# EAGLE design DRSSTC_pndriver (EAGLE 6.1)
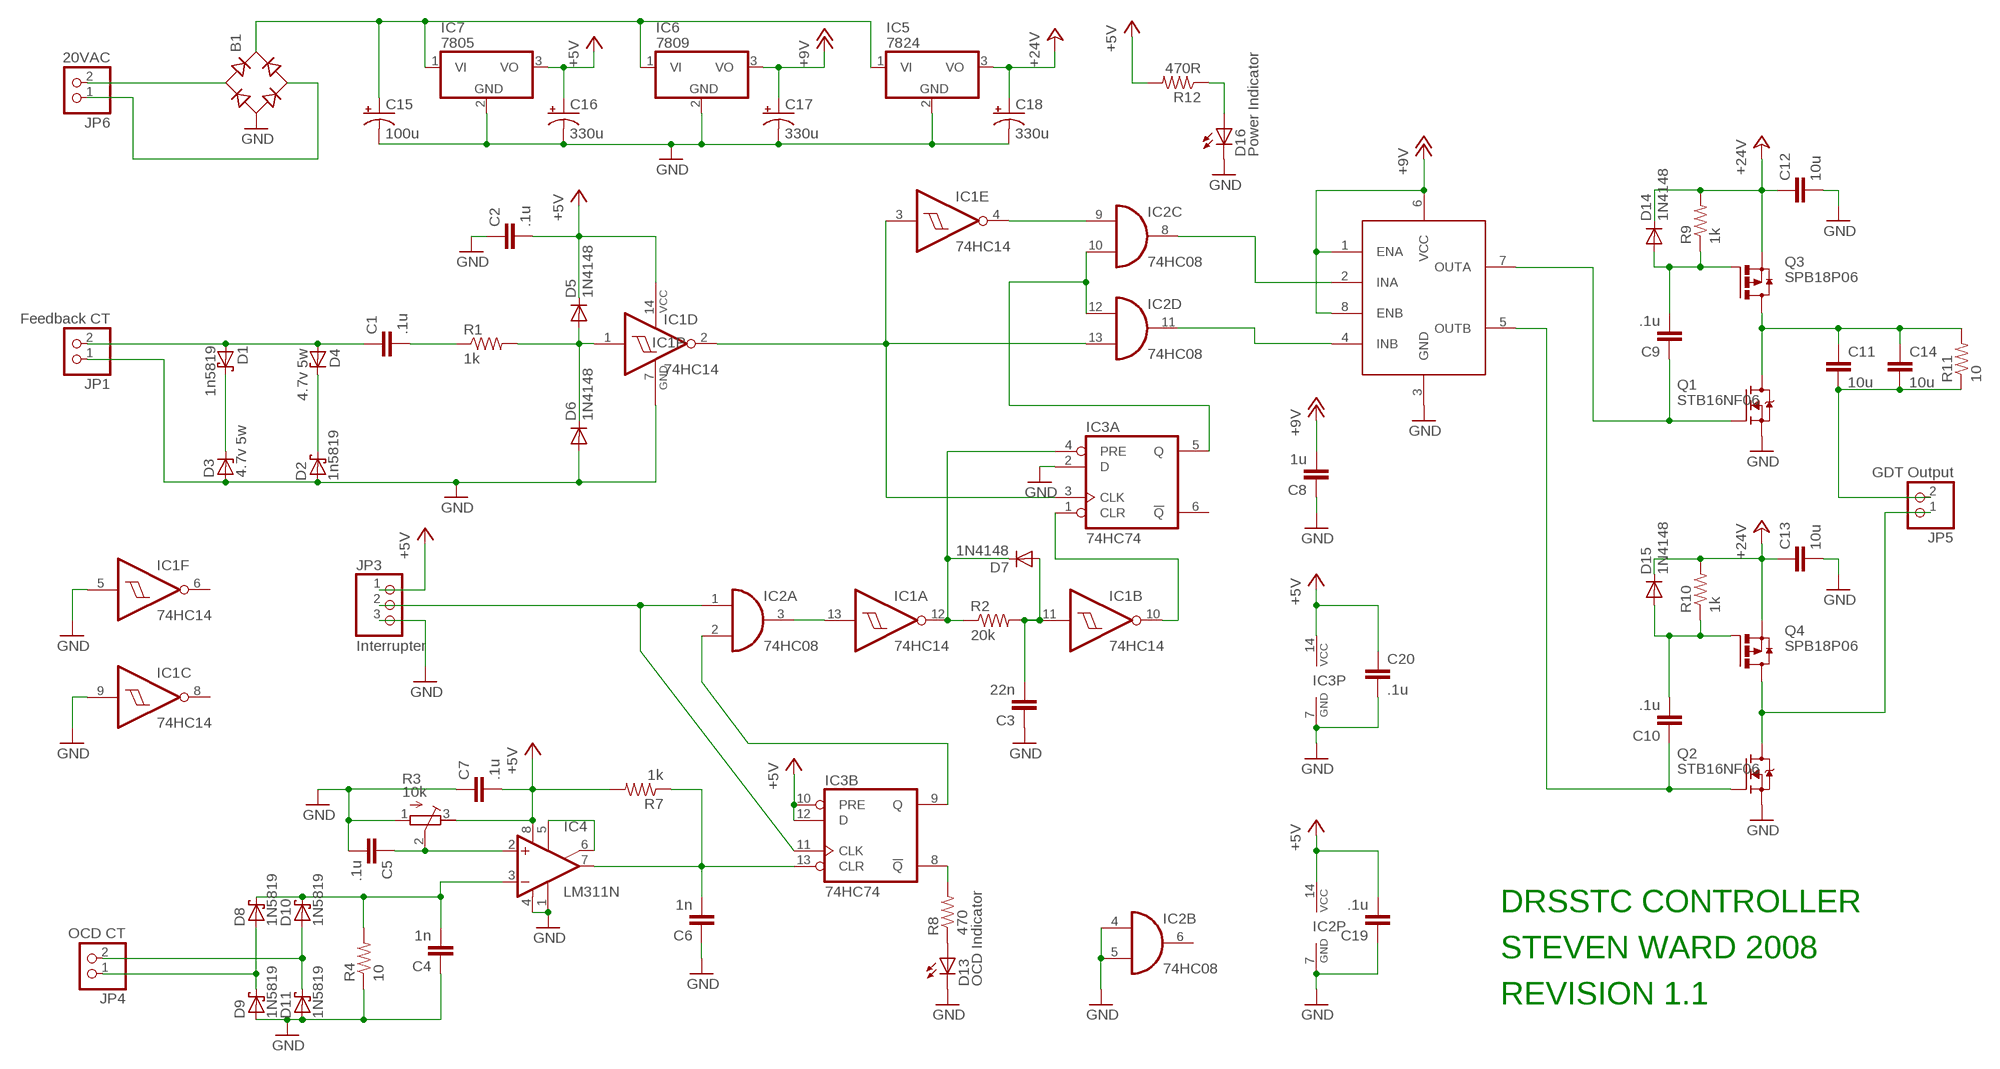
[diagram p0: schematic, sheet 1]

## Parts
B1  RB1A  [RB1A]
C1  .1u  C-EUC0805  [C0805]
C2  .1u  C-EUC0805  [C0805]
C3  22n  C-EUC0805  [C0805]
C4  1n  C-EUC0805  [C0805]
C5  .1u  C-EUC0805  [C0805]
C6  1n  C-EUC0805  [C0805]
C7  .1u  C-EUC0805  [C0805]
C8  1u  C-EUC0805  [C0805]
C9  .1u  C-EUC0805  [C0805]
C10  .1u  C-EUC0805  [C0805]
C11  10u  C-EUC1206  [C1206]
C12  10u  C-EUC1206  [C1206]
C13  10u  C-EUC1206  [C1206]
C14  10u  C-EUC1206  [C1206]
C15  100u  CPOL-USE5-10.5  [E5-10,5]
C16  330u  CPOL-USE5-10.5  [E5-10,5]
C17  330u  CPOL-USE5-10.5  [E5-10,5]
C18  330u  CPOL-USE5-10.5  [E5-10,5]
C19  .1u  C-EUC0805  [C0805]
C20  .1u  C-EUC0805  [C0805]
D1  1n5819  1N5819-BRADIAL  [C1702-05]
D2  1n5819  1N5819-BRADIAL  [C1702-05]
D3  4.7v 5w  ZENER-DIODEZD-5  [ZDIO-5]
D4  4.7v 5w  ZENER-DIODEZD-5  [ZDIO-5]
D5  1N4148  1N4148DO35-7  [DO35-7]
D6  1N4148  1N4148DO35-7  [DO35-7]
D7  1N4148  1N4148DO35-7  [DO35-7]
D8  1N5819  1N5819-BRADIAL  [C1702-05]
D9  1N5819  1N5819-BRADIAL  [C1702-05]
D10  1N5819  1N5819-BRADIAL  [C1702-05]
D11  1N5819  1N5819-BRADIAL  [C1702-05]
D13  OCD Indicator  SFH482  [SFH482]
D14  1N4148  1N4148DO35-7  [DO35-7]
D15  1N4148  1N4148DO35-7  [DO35-7]
D16  Power Indicator  SFH482  [SFH482]
IC1  74HC14  7414N  [DIL14]
IC2  74HC08  74HC08N  [DIL14]
IC3  74HC74  74HC74N  [DIL14]
IC4  LM311N  [DIL08]
IC5  7824  7824TV  [TO220V]
IC6  7809  L7809ACV  [TO220V]
IC7  7805  7805TV  [TO220V]
JP1  Feedback CT  PINHD-1X2  [1X02]
JP3  Interrupter  PINHD-1X3  [1X03]
JP4  OCD CT  PINHD-1X2  [1X02]
JP5  GDT Output  PINHD-1X2  [1X02]
JP6  20VAC  PINHD-1X2  [1X02]
Q1  STB16NF06  [D2PAK]
Q2  STB16NF06  [D2PAK]
Q3  SPB18P06  [D2PAK]
Q4  SPB18P06  [D2PAK]
R1  1k  R-US_M0805  [M0805]
R2  20k  R-US_M0805  [M0805]
R3  10k  R-TRIMM64W  [RTRIM64W]
R4  10  R-US_0617/5V  [0617V]
R7  1k  R-US_M0805  [M0805]
R8  470  R-US_M0805  [M0805]
R9  1k  R-US_M0805  [M0805]
R10  1k  R-US_M0805  [M0805]
R11  10  R-US_0617/5V  [0617V]
R12  470R  R-US_M0805  [M0805]
U1  UCC27423  [DIL08]

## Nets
+5V: C2.2 C7.2 C16.+ C19.2 C20.1 D5.C IC1.14(P:VCC) IC2.14(P:VCC) IC3.10(B:PRE) IC3.12(B:D) IC3.14(P:VCC) IC4.8(V+) IC7.3(VO) JP3.1 R3.3(E) R7.2 R12.2
+12V: C8.2 C17.+ IC6.3(VO) U1.1(ENA) U1.6(VCC) U1.8(ENB) ; supply symbol labelled +9V
+24V: C12.1 C13.1 C18.+ D14.C D15.C IC5.3(VO) Q3.3(S) Q4.3(S) R9.2 R10.2
GND: B1.- C2.1 C3.1 C4.1 C5.2 C6.1 C7.1 C8.1 C12.2 C13.2 C15.- C16.- C17.- C18.- C19.1 C20.2 D2.A D3.A D6.A D9.A D11.A D13.K(C) D16.K(C) IC1.5(F:I) IC1.7(P:GND) IC1.9(C:I) IC2.4(B:I0) IC2.5(B:I1) IC2.7(P:GND) IC3.2(A:D) IC3.7(P:GND) IC4.1(GND) IC4.4(V-) IC5.2(GND) IC6.2(GND) IC7.2(GND) JP1.1 JP3.3 Q1.3(S) Q2.3(S) R3.1(A) R4.1 U1.3(GND)
N$1: C1.1 D1.A D4.A JP1.2
N$2: C1.2 R1.1
N$3: D5.A D6.C IC1.1(D:I) R1.2
N$4: IC1.2(D:O) IC1.3(E:I) IC2.13(D:I1) IC3.3(A:CLK)
N$5: D2.C D4.C
N$6: D1.C D3.C
N$7: IC1.4(E:O) IC2.9(C:I0)
N$8: IC2.10(C:I1) IC2.12(D:I0) IC3.5(A:Q)
N$9: D13.A R8.1
N$10: IC3.8(B:!Q) R8.2
N$11: IC2.1(A:I0) IC3.11(B:CLK) JP3.2
N$12: IC2.2(A:I1) IC3.9(B:Q)
N$15: IC4.5(ON) IC4.6(ON/STR)
N$16: D7.C IC1.12(A:O) IC3.4(A:PRE) R2.1
N$17: C3.2 D7.A IC1.11(B:I) R2.2
N$18: IC1.10(B:O) IC3.1(A:CLR)
N$19: C9.1 Q1.1(G) U1.7(OUTA)
N$20: IC1.13(A:I) IC2.3(A:O)
N$21: C5.1 IC4.2(+IN) R3.2(S)
N$24: C4.2 D8.C D10.C IC4.3(-IN) R4.2
N$25: B1.AC1 JP6.2
N$26: IC2.11(D:O) U1.4(INB)
N$27: IC2.8(C:O) U1.2(INA)
N$28: C9.2 D14.A Q3.1(G) R9.1
N$29: B1.AC2 JP6.1
N$30: C11.1 C14.1 Q1.2(D) Q3.2(D) R11.2
N$31: C6.2 IC3.13(B:CLR) IC4.7(OUT) R7.1
N$32: B1.+ C15.+ IC5.1(VI) IC6.1(VI) IC7.1(VI)
N$33: C10.1 Q2.1(G) U1.5(OUTB)
N$34: C10.2 D15.A Q4.1(G) R10.1
N$35: D10.A D11.C JP4.2
N$36: D8.A D9.C JP4.1
N$37: JP5.1 Q2.2(D) Q4.2(D)
N$38: C11.2 C14.2 JP5.2 R11.1
N$41: D16.A R12.1
Unconnected: IC1.6(F:O) IC1.8(C:O) IC2.6(B:O) IC3.6(A:!Q)

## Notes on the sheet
- DRSSTC CONTROLLER
- STEVEN WARD 2008
- REVISION 1.1

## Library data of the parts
B1 = rectifier:RB1A: RECTIFIER 1 A
C1-C14 C19 C20 = rcl:C-EU: CAPACITOR, European symbol
C15-C18 = rcl:CPOL-US: POLARIZED CAPACITOR, American symbol
D1 D2 D8-D11 = diode:1N581*: 1.0A SCHOTTKY BARRIER RECTIFIER
D3 D4 = diode:ZENER-DIODE: Z-Diode
D5-D7 D14 D15 = diode:1N4148: DIODE
D13 D16 = led:SFH482: IR LED
IC1 = 74xx-us:74*14: Hex schmitt trigger INVERTER
IC2 = 74xx-eu:74*08: Quad 2-input AND gate
IC3 = 74xx-eu:74*74: Dual D type positive edge triggered FLIP FLOP, preset and clear
IC4 = linear:LM311: COMPARATOR
IC5 IC7 = linear:78*: Positive VOLTAGE REGULATOR Source: http://cache.national.com/ds/LM/LM78L05.pdf http://www.fairchildsemi.com/ds/LM/LM7805.pdf
IC6 = linear:L7809ACV
JP1 JP4-JP6 = pinhead:PINHD-1X2: PIN HEADER
JP3 = pinhead:PINHD-1X3: PIN HEADER
Q1 Q2 = uzzors2k:STB16NF06
Q3 Q4 = uzzors2k:SPB18P06
R1 R2 R4 R7-R12 = rcl:R-US_: RESISTOR, American symbol
R3 = rcl:R-TRIMM: Trimm resistor
U1 = uzzors2k:UCC27423

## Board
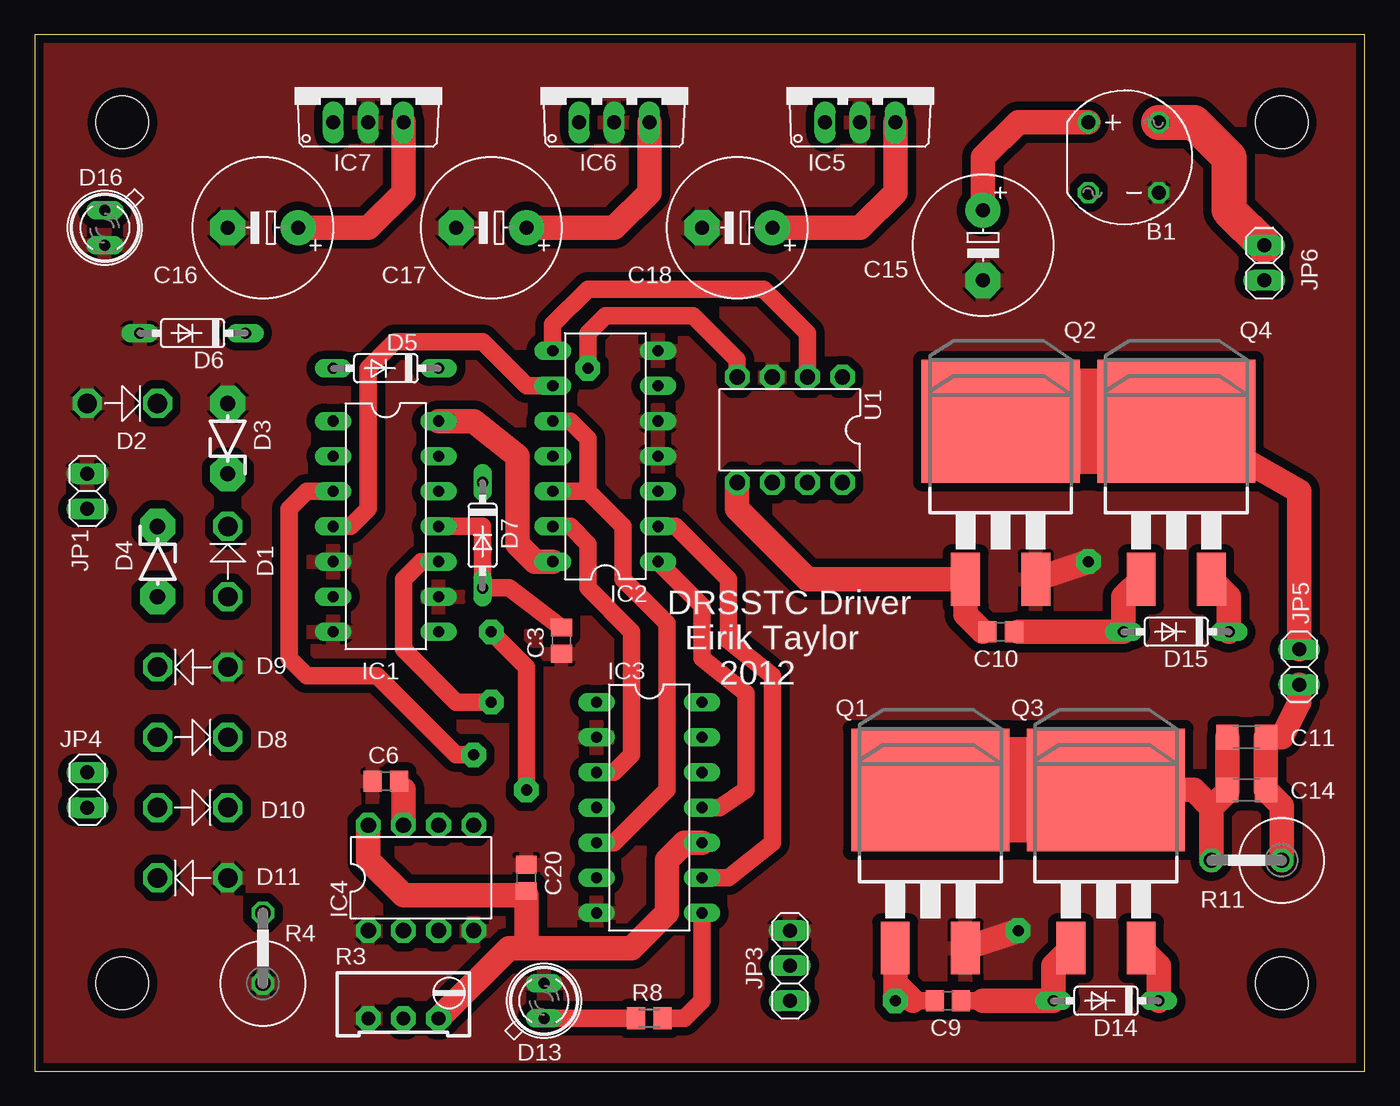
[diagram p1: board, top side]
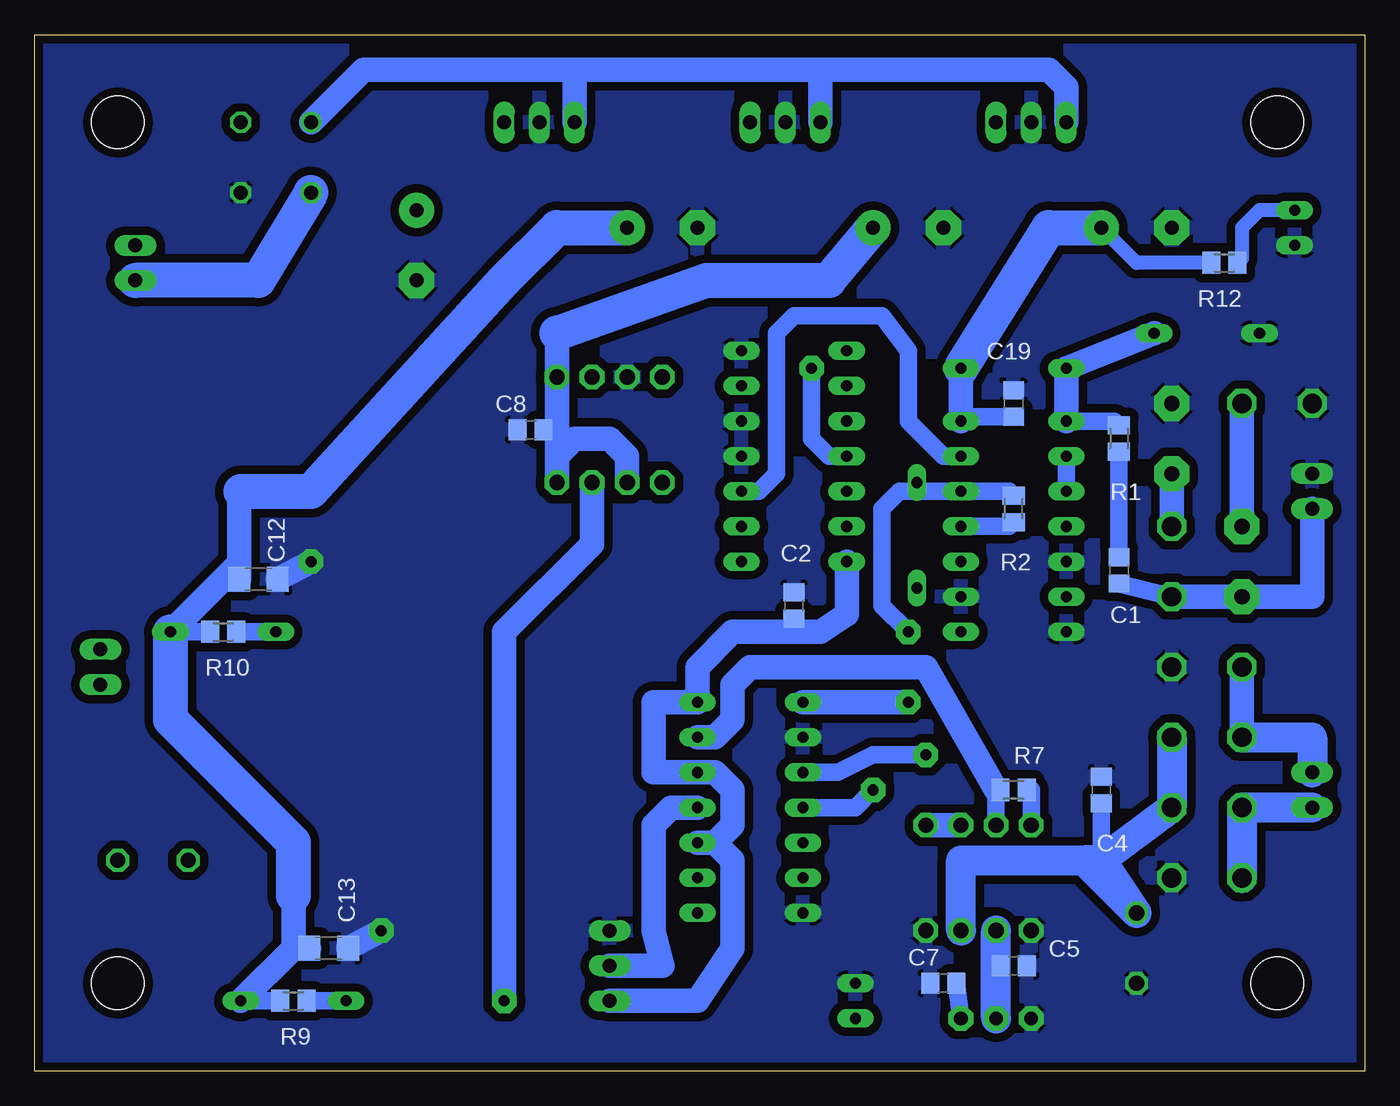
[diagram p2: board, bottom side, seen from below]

Size 96.19 x 74.92 mm. Coordinates in mm from the lower left corner, seen from the top.
Outline: 0,0 96.19,0 96.19,74.92 0,74.92 0,0
Copper layers (1*16): Top 0.035mm / dielectric 1.5mm / Bottom 0.035mm
Design rules: minimum track width 6mil, minimum drill 12mil, track to track 6mil, track to pad 6mil, pad to pad 6mil, via to via 6mil, smd to smd 0mil, copper to edge 10mil, drill to drill 10mil, minimum pad ring 10mil, minimum via ring 6mil, stop-mask expansion 2mil, vias tented up to drill 100mil, thermal gap 10mil
Holes 3.81 mm at 6.35,68.58 6.35,6.35 90.17,6.35 90.17,68.58

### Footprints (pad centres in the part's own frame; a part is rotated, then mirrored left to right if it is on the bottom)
RB1A = drill 1.016: + -2.54,2.54 | drill 1.016 octagon: - 2.54,-2.54; AC1 2.54,2.54; AC2 -2.54,-2.54
C0805 = smd 1.3 x 1.5: 1 -0.95,0; 2 0.95,0
C1206 = smd 1.6 x 1.8: 1 -1.4,0; 2 1.4,0
E5-10,5 = drill 1.016 pad 2.54: + -2.54,0 | drill 1.016 pad 2.54 octagon: - 2.54,0
C1702-05 = drill 1.397 octagon: A 2.54,0; C -2.54,0
ZDIO-5 = drill 1.1 pad 2.54 octagon: A 2.54,0; C -2.54,0
DO35-7 = drill 0.813 long: A 3.81,0; C -3.81,0
SFH482 = drill 0.813 long: A -1.27,0; K 1.27,0
DIL14 = drill 0.813 long: 1 -7.62,-3.81; 2 -5.08,-3.81; 3 -2.54,-3.81; 4 0,-3.81; 5 2.54,-3.81; 6 5.08,-3.81; 7 7.62,-3.81; 8 7.62,3.81; 9 5.08,3.81; 10 2.54,3.81; 11 0,3.81; 12 -2.54,3.81; 13 -5.08,3.81; 14 -7.62,3.81
DIL08 = drill 1.1 pad 1.778 octagon: 1 -3.81,-3.81; 2 -1.27,-3.81; 3 1.27,-3.81; 4 3.81,-3.81; 5 3.81,3.81; 6 1.27,3.81; 7 -1.27,3.81; 8 -3.81,3.81
TO220V = drill 1.016 long: 1 -2.54,-2.54; 2 0,-2.54; 3 2.54,-2.54
1X02 = drill 1.016 long: 1 -1.27,0; 2 1.27,0
1X03 = drill 1.016 long: 1 -2.54,0; 2 0,0; 3 2.54,0
D2PAK = smd 2.083 x 3.81: 1 -2.54,-10.16; 3 2.54,-10.16 | smd 11.43 x 8.89: 2 0,1.27
M0805 = smd 1.3 x 1.6: 1 -0.95,0; 2 0.95,0
RTRIM64W = drill 1 pad 1.778 octagon: 1 1.27,-2.54; 2 1.27,0; 3 1.27,2.54
0617V = drill 1.1 octagon: 1 -2.54,0; 2 2.54,0

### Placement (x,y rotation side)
B1  78.74,66.04 0 top
C1  17.78,36.2 90 bottom
C2  41.27,33.66 270 bottom
C3  38.1,31.11 90 top
C4  19.05,20.32 270 bottom
C5  25.4,7.62 0 bottom
C6  25.4,20.95 0 top
C7  30.48,6.35 0 bottom
C8  60.33,46.35 0 bottom
C9  66.04,5.08 0 top
C10  69.85,31.75 0 top
C11  87.63,24.13 0 top
C12  80.01,35.56 0 bottom
C13  74.93,8.89 0 bottom
C14  87.63,20.32 0 top
C15  68.58,59.69 270 top
C16  16.51,60.96 180 top
C17  33.02,60.96 180 top
C18  50.8,60.96 180 top
C19  25.4,48.26 270 bottom
C20  35.56,13.97 90 top
D1  13.97,36.83 270 top
D2  6.35,48.26 180 top
D3  13.97,45.72 90 top
D4  8.89,36.83 270 top
D5  25.4,50.8 180 top
D6  11.43,53.34 180 top
D7  32.38,38.73 270 top
D8  11.43,24.13 180 top
D9  11.43,29.21 0 top
D10  11.43,19.05 180 top
D11  11.43,13.97 0 top
D13  36.83,5.08 90 top
D14  77.47,5.08 180 top
D15  82.55,31.75 180 top
D16  5.08,60.96 270 top
IC1  25.4,39.37 270 top
IC2  41.27,44.45 90 top
IC3  44.45,19.05 270 top
IC4  27.94,13.97 0 top
IC5  59.69,71.12 0 top
IC6  41.91,71.12 0 top
IC7  24.13,71.12 0 top
JP1  3.81,41.91 270 top
JP3  54.61,7.62 90 top
JP4  3.81,20.32 270 top
JP5  91.44,29.21 270 top
JP6  88.9,58.42 90 top
Q1  64.77,19.05 0 top
Q2  69.85,45.72 0 top
Q3  77.47,19.05 0 top
Q4  82.55,45.72 0 top
R1  17.78,45.72 90 bottom
R2  25.4,40.64 270 bottom
R3  26.67,5.08 270 top
R4  16.51,8.89 90 top
R7  25.4,20.32 0 bottom
R8  44.45,3.81 0 top
R9  77.47,5.08 180 bottom
R10  82.55,31.75 180 bottom
R11  87.63,15.24 180 top
R12  10.16,58.42 180 bottom
U1  54.61,46.35 180 top

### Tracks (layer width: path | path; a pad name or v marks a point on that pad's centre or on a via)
+5V
  Top 1.27: C20.1 35.56,12.7
  Top 1.778: IC4.8 24.13,15.24 26.67,12.7 35.56,12.7 35.56,8.89 | IC3.10 46.99,16.51 45.72,15.24 45.72,11.43 43.18,8.89 35.56,8.89 | IC2.14 36.2,36.83 34.92,38.1 34.92,44.45 31.75,46.99 IC1.14 | IC7.3 26.67,63.5 24.13,60.96 C16.+ | 35.56,8.89 34.29,8.89 R3.3
  Bottom 1.016: R12.2 16.51,58.42 C16.+
  Bottom 1.27: C7.2 R3.3 | R7.2 24.13,20.32 IC4.8 | C19.2 28.89,47.31 IC1.14 | C2.2 41.27,31.75
  Bottom 1.778: JP3.1 48.26,5.08 45.72,8.89 45.72,15.24 46.99,16.51 | 46.99,16.51 IC3.10 | 46.99,16.51 45.72,17.78 45.72,20.32 46.99,21.59 IC3.12 51.44,21.59 51.44,26.67 IC3.14 48.26,29.21 45.72,31.75 41.27,31.75 39.37,31.75 37.47,33.02 IC2.14 | D5.C IC1.14
  Bottom 2.54: D5.C 22.86,60.96 C16.+
+12V
  Top 1.778: C17.+ 41.91,60.96 44.45,63.5 IC6.3
  Bottom 1.27: C8.2 58.42,46.35
  Bottom 1.778: U1.6 53.34,44.45 54.61,45.72 57.15,45.72 58.42,44.45 | 58.42,44.45 U1.8 | 58.42,44.45 58.42,46.35 U1.1 58.42,53.34
  Bottom 2.54: 58.42,53.34 47.62,57.15 38.73,57.15 C17.+
+24V
  Top 1.778: D14.C 81.28,7.62 Q3.3 | Q4.3 86.36,34.29 D15.C | C18.+ 59.69,60.96 62.23,63.5 IC5.3
  Bottom 1.27: R10.2 D15.C | R9.2 D14.C
  Bottom 1.778: D15.C 81.41,36.7 C12.1 81.41,41.78 81.28,41.91 | C13.1 77.47,8.89 | 77.47,8.89 77.47,12.7 | 77.47,8.89 D14.C
  Bottom 2.54: 81.28,41.91 76.2,41.91 62.23,57.15 58.42,60.96 C18.+ | 77.47,12.7 77.47,16.51 86.36,25.4 D15.C
GND  (via drill 0.8 pad 1.78)
  Top 1.778: v76.2,36.83 Q2.3 | Q1.3 v71.12,10.16
  Bottom 1.778: C12.2 v76.2,36.83 | v71.12,10.16 C13.2
  pour Bottom (isolate 0.61): 0,74.93 100.33,74.93 100.33,0 0,0
  pour Top (isolate 0.61): 0,74.93 105.41,74.93 105.41,0 0,0
N$1
  Bottom 1.27: C1.1 D1.A
  Bottom 1.778: JP1.2 3.81,34.29 D4.A D1.A
N$2
  Bottom 1.27: R1.1 C1.2
N$3
  Bottom 1.27: IC1.1 18.1,46.99 R1.2
  Bottom 1.778: IC1.1 D5.A D6.C
N$4  (via drill 0.8 pad 1.78)
  Top 1.27: IC3.3 41.91,21.59 43.18,22.86 43.18,31.75 40.01,34.92 40.01,38.1 38.73,39.37 IC2.13 | IC1.3 19.68,41.91 18.41,40.64 18.41,29.84 19.68,28.57 24.77,28.57 30.48,22.86 v31.75,22.86
  Bottom 1.27: IC1.2 IC1.3 | v31.75,22.86 35.56,22.86 38.1,21.59 IC3.3
N$5
  Bottom 1.778: D4.C D2.C
N$6
  Bottom 1.778: D3.C D1.C
N$7
  Top 1.27: IC2.9 35.56,49.53 32.38,52.7 26.04,52.7 24.13,50.8 24.13,40.64 22.86,39.37 IC1.4
N$8
  Top 1.27: IC3.5 41.91,16.51 45.72,20.32 45.72,32.38 42.55,35.56 42.55,39.37 40.01,41.91 | 40.01,41.91 IC2.12 | IC2.10 38.73,46.99 40.01,45.72 40.01,41.91
N$9
  Top 1.27: R8.1 D13.A
N$10
  Top 1.27: R8.2 46.99,3.81 48.26,5.08 IC3.8
N$11
  Top 1.27: IC3.11 49.53,19.05 51.44,20.32 51.44,27.3 48.26,29.84 48.26,33.66 IC2.1
  Bottom 1.778: IC3.11 50.16,19.05 51.44,17.78 51.44,10.16 50.8,7.62 JP3.2
N$12
  Top 1.27: IC3.9 50.16,13.97 53.34,16.51 53.34,28.57 50.16,31.11 50.16,35.56 46.35,39.37 IC2.2
N$15
  Bottom 1.778: IC4.6 IC4.5
N$16  (via drill 0.8 pad 1.78)
  Top 1.27: v35.56,20.32 35.56,29.21 v33.02,31.75
  Bottom 1.27: IC3.4 36.83,19.05 v35.56,20.32 | R2.1 25.72,41.91 IC1.12 32.38,41.91 | v33.02,31.75 34.92,33.66 34.92,40.64 33.66,41.91 32.38,41.91 | D7.C 32.38,41.91
N$17
  Top 1.27: IC1.11 32.38,39.37 D7.A 34.29,34.92 C3.2
  Bottom 1.27: IC1.11 25.72,39.37 R2.2
N$18  (via drill 0.8 pad 1.78)
  Top 1.27: v33.02,26.67 30.48,26.67 26.67,30.48 26.67,35.56 27.94,36.83 IC1.10
  Bottom 1.778: IC3.1 v33.02,26.67
N$19  (via drill 0.8 pad 1.78)
  Top 1.27: C9.1 63.5,5.08
  Top 1.778: 63.5,5.08 62.23,6.35 Q1.1 v62.23,5.08
  Bottom 1.778: v62.23,5.08 62.23,31.75 55.88,38.1 U1.7
N$20
  Bottom 1.27: IC1.13 30.48,44.45 33.02,46.99 33.02,52.07 34.92,54.61 41.27,54.61 42.55,53.34 42.55,43.18 43.81,41.91 IC2.3
N$21
  Bottom 1.27: C5.1 26.35,9.84 IC4.2
  Bottom 2.184: R3.2 IC4.2
N$24
  Bottom 1.27: C4.2 19.05,15.24
  Bottom 2.184: D8.C D10.C 19.05,15.24 | 19.05,15.24 R4.2 20.32,15.24 | IC4.3 29.21,15.24 20.32,15.24 | 19.05,15.24 20.32,15.24
N$25
  Top 2.54: B1.AC1 83.82,68.58 86.36,66.04 86.36,62.23 JP6.2
N$26  (via drill 0.8 pad 1.78)
  Top 1.27: v40.01,50.8 40.01,53.34 41.27,54.61 47.62,54.61 50.8,51.44 U1.4
  Bottom 1.27: IC2.11 38.73,44.45 40.01,45.72 v40.01,50.8
N$27
  Top 1.27: IC2.8 37.47,53.98 40.01,56.52 52.7,56.52 55.88,53.34 U1.2
N$28
  Top 1.27: C9.2 68.58,5.08
  Top 1.778: Q3.1 73.66,7.62 D14.A 68.58,5.08
  Bottom 1.27: R9.1 D14.A
N$29
  Bottom 2.54: B1.AC2 80.01,57.15 JP6.1
N$30
  Top 1.778: C11.1 C14.1 86.23,20.19 85.09,19.05 | 85.09,19.05 R11.2 | Q3.2 83.82,20.32 85.09,19.05
  Top 7.62: Q1.2 Q3.2
N$31
  Top 1.27: C6.2 26.35,20.64 26.67,20.32
  Top 1.778: 26.67,20.32 IC4.7
  Bottom 1.27: R7.1 26.67,20.32 IC4.7
  Bottom 1.778: IC3.13 46.99,24.13 45.72,25.4 45.72,27.94 44.45,29.21 31.75,29.21 26.67,20.32
N$32
  Top 1.778: C15.+ 68.58,66.04 71.12,68.58 B1.+
  Bottom 1.778: IC7.1 21.59,71.12 22.86,72.39 39.37,72.39 | 39.37,72.39 57.15,72.39 | 57.15,72.39 72.39,72.39 B1.+ | IC5.1 57.15,72.39 | IC6.1 39.37,72.39
N$33
  Top 1.27: 68.58,31.75 C10.1
  Top 1.778: 68.58,31.75 67.31,33.02 Q2.1 55.88,35.56 50.8,40.64 U1.5
N$34
  Top 1.27: 71.12,31.75 C10.2
  Top 1.778: Q4.1 78.74,34.29 D15.A 71.12,31.75
  Bottom 1.27: R10.1 D15.A
N$35
  Bottom 2.184: JP4.2 D10.A D11.C
N$36
  Bottom 1.778: D8.A D9.C
  Bottom 2.184: D8.A 3.81,24.13 JP4.1
N$37
  Top 1.778: Q4.2 91.44,41.91 JP5.1
  Top 7.62: Q2.2 Q4.2
N$38
  Top 1.778: R11.1 90.17,19.18 C14.2 C11.2 90.17,24.13 91.44,26.67 JP5.2
N$41
  Bottom 1.016: D16.A 7.62,62.23 8.89,60.96 8.89,58.74 R12.1

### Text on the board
tPlace: DRSSTC Driver | Eirik Taylor | 2012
